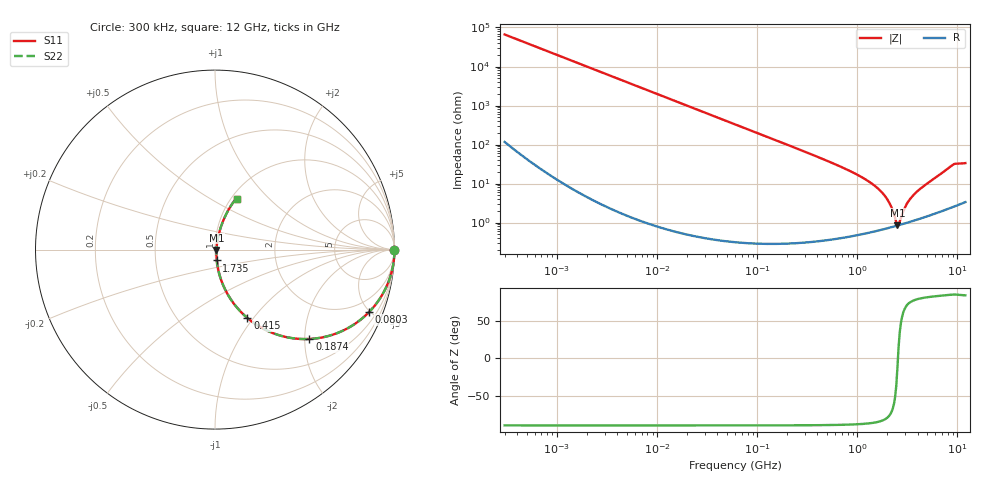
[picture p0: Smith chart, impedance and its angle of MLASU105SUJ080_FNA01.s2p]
! MLASU105SUJ080_FNA01  S-PARAMETER MODEL  ( General Type )
! Model Generated by TAIYO YUDEN Corporation (http://www.ty-top.com)
! Version 3.0
! TAIYO YUDEN Control No. 121128
! Copyright(c) 2011 TAIYO YUDEN CO.,LTD. All Rights Reserved.
! Product Description (link to TY-COMPAS)
! https://ds.yuden.co.jp/TYCOMPAS/or/detail?pn=MLASU105SUJ080DFNA01&u=M
! Products Name : Multilayer Ceramic Capacitors
! Characteristics :
!  Capacitance : 8 pF , Rated Voltage : 50V , TCC : UJ / U2J
!  Case Size : 1.0 x 0.5 / 0.039 x 0.02 [mm/inch] , Thickness : 0.5 / 0.02 [mm/inch]
!  (Conditions: Temperature = 25 degC , DC Bias Current/Voltage = 0A / 0V)
! External Node Assignments :
!  1  o---| |---o  2
! GND o---------o GND
! Frequency Range : 300000Hz  -  12GHz  [ 401 STEP ]
# MHz S RI R 50
! Freq[MHz].  S11 Real  S11 Imag  S21 Real  S21 Imag  S12 Real  S12 Imag  S22 Real  S22 Imag
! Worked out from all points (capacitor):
!   401 points, 300 kHz to 12 GHz, reference 50 ohm
!   read as one part in series: C = 8.01 pF near 316.3 kHz
!   lowest |Z| = 860 mohm at 2.514 GHz (marker M1)
!   series resonance near 2.545 GHz, so ESL is about 490 pH
!   S11 on the Smith chart (normalised r, x): 300 kHz: open; 80.3 MHz: 1.01, -4.94; 187.4 MHz: 1.01, -2.11; 415 MHz: 1.01, -0.93; 1.735 GHz: 1.01, -0.12; 12 GHz: 1.07, +0.67
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0.3  1 -0.00151  4.94e-06 0.00151  4.94e-06 0.00151  1 -0.00151
1.769972  0.9999 -0.00891  8.36e-05 0.00891  8.36e-05 0.00891  0.9999 -0.00891
10.44266  0.9972 -0.0524  0.00278 0.0524  0.00278 0.0524  0.9972 -0.0524
27.10171  0.9817 -0.1339  0.0183 0.1339  0.0183 0.1339  0.9817 -0.1339
60  0.9161 -0.2767  0.0839 0.2767  0.0839 0.2767  0.9161 -0.2767
80.29859  0.8591 -0.3473  0.1409 0.3473  0.1409 0.3473  0.8591 -0.3473
119.4772  0.7332 -0.4414  0.2668 0.4414  0.2668 0.4414  0.7332 -0.4414
187.4445  0.5263 -0.4979  0.4737 0.4979  0.4737 0.4979  0.5263 -0.4979
353.9943  0.2339 -0.4204  0.7661 0.4204  0.7661 0.4204  0.2339 -0.4204
414.98  0.1802 -0.3808  0.8198 0.3808  0.8198 0.3808  0.1802 -0.3808
1021.415  0.0304 -0.1575  0.9696 0.1575  0.9696 0.1575  0.0304 -0.1575
1403.667  0.0151 -0.0965  0.9849 0.0965  0.9849 0.0965  0.0151 -0.0965
1735.023  0.0102 -0.0603  0.9898 0.0603  0.9898 0.0603  0.0102 -0.0603
2088.533  0.00826 -0.0307  0.9917 0.0307  0.9917 0.0307  0.00826 -0.0307
2448.343  0.0082 -0.00607  0.9918 0.00607  0.9918 0.00607  0.0082 -0.00607
2514.07  0.00832 -0.00185  0.9917 0.00185  0.9917 0.00185  0.00832 -0.00185
2650.866  0.00868 0.0059  0.9913 -0.0059  0.9913 -0.0059  0.00868 0.0059
2947.191  0.00975 0.02  0.9903 -0.02  0.9903 -0.02  0.00975 0.02
3276.641  0.0113 0.0344  0.9887 -0.0344  0.9887 -0.0344  0.0113 0.0344
4050.141  0.016 0.0633  0.984 -0.0633  0.984 -0.0633  0.016 0.0633
8966.534  0.101 0.2626  0.899 -0.2626  0.899 -0.2626  0.101 0.2626
12000  0.1235 0.2826  0.8765 -0.2826  0.8765 -0.2826  0.1235 0.2826
